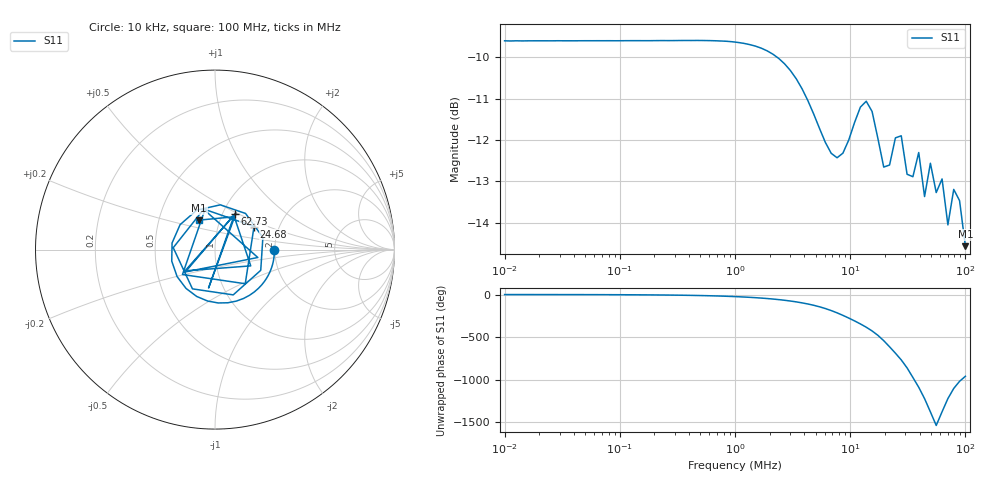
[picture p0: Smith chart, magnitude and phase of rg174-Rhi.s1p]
! ListType=Log
!!RG174 24.9f Rhi
# MHz S RI R 50
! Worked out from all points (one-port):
!   80 points, 10 kHz to 100 MHz, reference 50 ohm
!   lowest |S11| = -14.6 dB at 100 MHz (marker M1), VSWR 1.46, Z = 39.8 + j13.5 ohm
!   |S11| at or under -10 dB: 2.323 MHz to end of sweep
!   S11 on the Smith chart (normalised r, x): 10 kHz: 1.99, -0.01; 24.68 MHz: 1.49, +0.41; 62.73 MHz: 1.14, +0.47; 100 MHz: 0.80, +0.27
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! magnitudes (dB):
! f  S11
! 10 kHz  -9.6
! 32.09 kHz  -9.6
! 103 kHz  -9.6
! 330.4 kHz  -9.6
! 1.06 MHz  -9.6
! 2.134 MHz  -9.9
! 3.401 MHz  -10.5
! 6.093 MHz  -12.1
! 7.693 MHz  -12.4
! 8.644 MHz  -12.3
! 10.91 MHz  -11.6
! 13.78 MHz  -11.1
! 15.48 MHz  -11.3
! 19.55 MHz  -12.7
! 21.97 MHz  -12.6
! 24.68 MHz  -11.9
! 27.74 MHz  -11.9
! 31.17 MHz  -12.8
! 35.02 MHz  -12.9
! 39.35 MHz  -12.3
! 44.21 MHz  -13.4
! 49.68 MHz  -12.6
! 55.83 MHz  -13.3
! 62.73 MHz  -12.9
! 70.49 MHz  -14.1
! 79.2 MHz  -13.2
! 89 MHz  -13.5
! 100 MHz  -14.6
